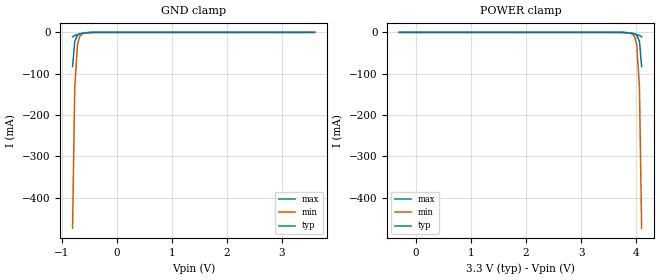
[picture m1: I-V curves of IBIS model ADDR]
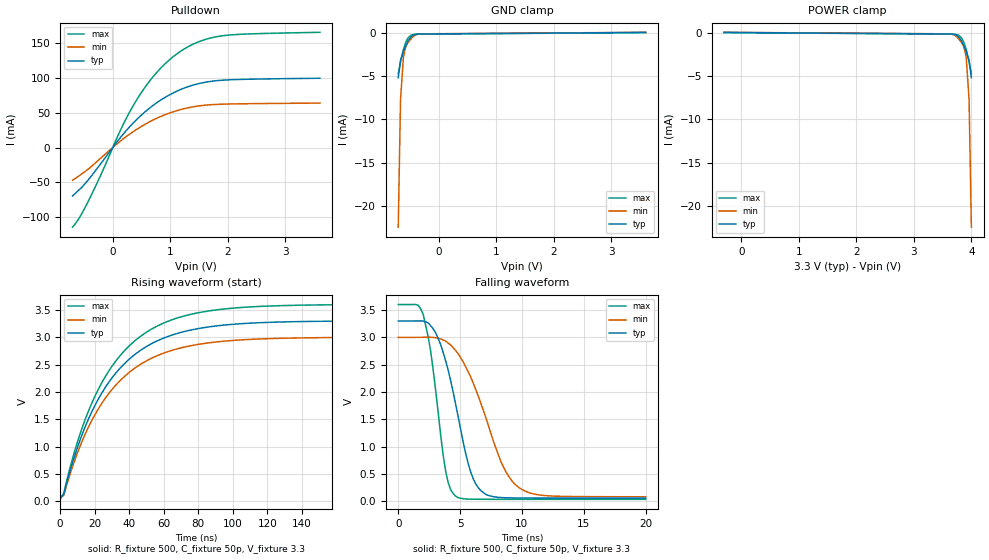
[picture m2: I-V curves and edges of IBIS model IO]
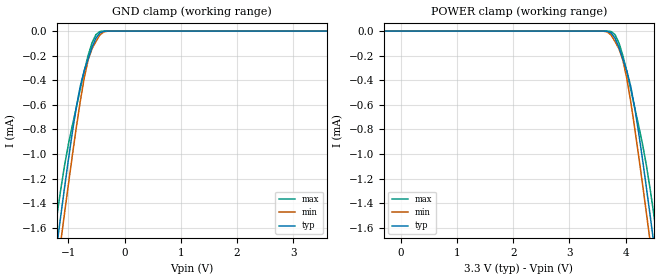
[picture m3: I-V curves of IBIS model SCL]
[IBIS Ver]   3.2
[Comment Char]   |_char
| Vnom = 3.3v, Vmin = 3v, Vmax = 3.6v
[File name]   pca8575_3_3v.ibs
[File Rev]   1
[Date]   Aug 6, 2008 4:45:34 PM
[Source]
Generated by Seshadri Venkataramanan using IBIS Toolkit at NXP Tempe
[Notes]
[Disclaimer]
(C) Copyright 2007 NXP Semiconductors
All rights reserved
NXP Semiconductors (NXP) does not warrant that this model and any other
accompanying information (Model) accurately or fully represents the
operating characteristics and specifications of the semiconductor
products to which the Model relates.  Moreover, the Model is furnished
on an "as is" and with "all faults" basis, and without support or
warranty of any kind.  NXP disclaims all warranties, whether expressed
or implied or statutory, including without limitation all implied
warranties of non-infringement, merchantability and fitness for any
purpose, and those arising from a course of dealing or usage of trade.
NXP does not convey any license under its or any third party's patents,
copyrights or other intellectual property or proprietary rights.
You and your company assume any and all risks and liability arising out
of the application or use of the Model.
In no event shall NXP be liable for any direct, indirect, special,
consequential or incidental damages, however caused, whether in
warranty, contract or tort (including negligence), strict liability or
other legal theory, including, without limitation, for lost profits,
business interruption, or corruption or loss of data or information,
arising out of or in connection with the use of or the inability to use
the Model, even if NXP has been advised of the possibility of such
damages.
NXP provides the Model as a courtesy to our customers. You and your
company shall not distribute, convey, sell, or give the Model to anyone
else without receiving prior written permission from NXP.
NXP reserves the right to make changes without notice to the Model to
improve reliability, function, or design.
Please be aware that your receipt and subsequent use of the Model shall
serve as acceptance of these terms and conditions.  If you do not
accept these terms, return or destroy the Model immediately.
[Copyright]
2008
| SO24 package
[Component]   PCA8575D
Si_location Pin
Timing_location Pin
[Manufacturer]   NXP Semiconductors
[Package]
R_pkg   0.14   0.12   0.18
L_pkg   5.71n   3.95n   7.95n
C_pkg   1.01p   0.72p   1.49p
[Pin] signal_name   model_name   R_pin   L_pin   C_pin
1   INTb   INT_OUT   0.18   6.01n   0.97p
2   AD1   ADDR   0.14   7.94n   1.21p
3   AD2   ADDR   0.16   7.06n   1.32p
4   P00   IO   0.18   6.01n   1.07p
5   P01   IO   0.14   4.98n   0.88p
6   P02   IO   0.13   4.30n   0.80p
7   P03   IO   0.12   3.95n   0.74p
8   P04   IO   0.12   3.95n   0.72p
9   P05   IO   0.13   4.30n   0.76p
10   P06   IO   0.14   4.98n   0.85p
11   P07   IO   0.18   6.01n   0.97p
12   VSS   GND   0.16   7.06n   1.20p
13   P10   IO   0.14   7.95n   1.45p
14   P11   IO   0.14   7.95n   1.49p
15   P12   IO   0.16   7.06n   1.32p
16   P13   IO   0.18   6.01n   1.07p
17   P14   IO   0.14   4.98n   0.88p
18   P15   IO   0.13   4.30n   0.80p
19   P16   IO   0.12   3.95n   0.74p
20   P17   IO   0.12   3.95n   0.72p
21   AD0   ADDR   0.13   4.30n   0.76p
22   SCL   SCL   0.14   4.98n   0.85p
23   SDA   SDAIO   0.18   6.01n   0.97p
24   VDD   POWER   0.16   7.06n   1.20p
| TSSOP24 package
[Component]   PCA8575PW
Si_location Pin
Timing_location Pin
[Manufacturer]   NXP Semiconductors
[Package]
R_pkg   52.70m   31.50m   67.00m
L_pkg   2.19n   1.32n   3.39n
C_pkg   0.48p   0.35p   0.93p
[Pin] signal_name   model_name   R_pin   L_pin   C_pin
1   INTb   INT_OUT   66.40m   2.36n   0.47p
2   AD1   ADDR   66.10m   3.39n   0.57p
3   AD2   ADDR   67.00m   2.94n   0.59p
4   P00   IO   66.40m   2.36n   0.47p
5   P01   IO   47.10m   1.67n   0.40p
6   P02   IO   38.00m   1.44n   0.37p
7   P03   IO   31.50m   1.32n   0.35p
8   P04   IO   31.50m   1.32n   0.35p
9   P05   IO   38.00m   1.44n   0.37p
10   P06   IO   47.10m   1.67n   0.40p
11   P07   IO   66.40m   2.36n   0.47p
12   VSS   GND   67.00m   2.94n   0.59p
13   P10   IO   66.10m   3.39n   0.61p
14   P11   IO   66.20m   3.39n   0.61p
15   P12   IO   67.00m   2.94n   0.59p
16   P13   IO   66.50m   2.36n   0.47p
17   P14   IO   47.10m   1.67n   0.40p
18   P15   IO   38.00m   1.45n   0.37p
19   P16   IO   31.50m   1.32n   0.35p
20   P17   IO   31.50m   1.32n   0.35p
21   AD0   ADDR   38.00m   1.45n   0.37p
22   SCL   SCL   47.10m   1.67n   0.40p
23   SDA   SDAIO   66.50m   2.36n   0.47p
24   VDD   POWER   67.00m   2.94n   0.59p
| SSOP24
[Component]   PCA8575DB
Si_location Pin
Timing_location Pin
[Manufacturer]   NXP Semiconductors
[Package]
R_pkg   54.20m   39.70m   64.80m
L_pkg   2.55n   1.89n   3.58n
C_pkg   0.636p   0.52p   1.05p
[Pin] signal_name   model_name   R_pin   L_pin   C_pin
1   INTb   INT_OUT   63.00m   2.53n   0.58p
2   AD1   ADDR   61.20m   3.56n   0.70p
3   AD2   ADDR   64.80m   3.10n   0.76p
4   P00   IO   63.00m   2.53n   0.60p
5   P01   IO   52.60m   2.17n   0.57p
6   P02   IO   43.90m   2.03n   0.56p
7   P03   IO   39.70m   1.89n   0.54p
8   P04   IO   39.70m   1.89n   0.52p
9   P05   IO   43.90m   2.03n   0.55p
10   P06   IO   52.60m   2.17n   0.56p
11   P07   IO   63.00m   2.53n   0.58p
12   VSS   GND   64.80m   3.10n   0.71p
13   P10   IO   61.20m   3.56n   1.01p
14   P11   IO   61.20m   3.56n   1.05p
15   P12   IO   64.80m   3.10n   0.80p
16   P13   IO   63.00m   2.53n   0.65p
17   P14   IO   52.60m   2.17n   0.59p
18   P15   IO   43.90m   2.03n   0.56p
19   P16   IO   39.70m   1.89n   0.54p
20   P17   IO   39.70m   1.89n   0.53p
21   AD0   ADDR   43.90m   2.03n   0.56p
22   SCL   SCL   52.60m   2.17n   0.57p
23   SDA   SDAIO   63.00m   2.53n   0.60p
24   VDD   POWER   64.80m   3.10n   0.76p
[Define Package Model]  HVQFN24
[Manufacturer]  ST-NXP Wireless
|[Simulated] Chris Hunat
|[Approved] Wayne Nunn, Roger Real
[OEM]  Unknown
[Description]  Full package model
[Number Of Pins]  23
[Pin Numbers]
pin1   | pin1 = lead1
pin2   | pin2 = lead2
pin3   | pin3 = lead3
pin4   | pin4 = lead4
pin5   | pin5 = lead5
pin6   | pin6 = lead6
pin7   | pin7 = lead7
pin8   | pin8 = lead8
pin9   | pin9 = lead9
pin10   | pin10 = lead10
pin11   | pin11 = lead11
pin12   | pin12 = lead12
pin13   | pin13 = lead13
pin14   | pin14 = lead14
pin15   | pin15 = lead15
pin17   | pin17 = lead17
pin18   | pin18 = lead18
pin19   | pin19 = lead19
pin20   | pin20 = lead20
pin21   | pin21 = lead21
pin22   | pin22 = lead22
pin23   | pin23 = lead23
pin24   | pin24 = lead24
[Model Data]
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[End Model Data]
[End Package Model]
[Define Package Model]  DHVQFN24
[Manufacturer]  ST-NXP Wireless
|[Simulated] Chris Hunat
|[Approved] Wayne Nunn, Roger Real
[OEM]  Unknown
[Description]  Full package model
[Number Of Pins]  24
[Pin Numbers]
|Pin Num   Terminal Name
1   | lead1:pin1
2   | lead2:pin2
3   | lead3:pin3
4   | lead4:pin4
5   | lead5:pin5
6   | lead6:pin6
7   | lead7:pin7
8   | lead8:pin8
9   | lead9:pin9
10   | lead10:pin10
11   | lead11:pin11
12   | lead12:pin12
13   | lead13:pin13
14   | lead14:pin14
15   | lead15:pin15
16   | lead16:pin16
17   | lead17:pin17
18   | lead18:pin18
19   | lead19:pin19
20   | lead20:pin20
21   | lead21:pin21
22   | lead22:pin22
23   | lead23:pin23
24   | lead24:pin24
[Model Data]
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[End Model Data]
[End Package Model]
| Models and submodels in the file (5): ADDR (Input), IO (I/O_open_drain), SCL (Input), SDAIO (I/O_open_drain), INT_OUT (Open_drain)
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[Model]   ADDR
Model_type Input
Vinh=2.31
Vinl=0.99
C_comp   0.73p   0.7p   0.76p
[Temperature Range] 27   85   -40
[Voltage Range]   3.3   3   3.6
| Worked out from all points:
|   GND clamp passes 1 mA (typ) near -0.54 V on its own axis
[GND Clamp]
-800mV    -82.74mA   -473.3mA   -10.75mA
-760mV    -21.49mA   -132.6mA   -7.457mA
-710mV    -6.279mA   -28.8mA    -5.482mA
-670mV    -3.609mA   -9.611mA   -3.955mA
-620mV    -2.373mA   -3.263mA   -2.228mA
-360mV    -13.44uA   -47.6uA    -1.436uA
3.6V      65.11pA    250.9pA    47.06pA
[POWER Clamp]
-300mV    65.11pA    250.9pA    47.06pA
3.66V     -13.44uA   -47.6uA    -1.436uA
3.92V     -2.373mA   -3.263mA   -2.228mA
3.97V     -3.609mA   -9.611mA   -3.955mA
4.01V     -6.279mA   -28.8mA    -5.482mA
4.06V     -21.49mA   -132.6mA   -7.457mA
4.1V      -82.74mA   -473.3mA   -10.75mA
[Model]   IO
Model_type I/O_open_drain
Vinh=2.31
Vinl=0.99
Vref=3.3
Vmeas=1.65
Rref=500
Cref=50p
C_comp   6.3p   6.1p   6.5p
[Temperature Range] 27   85   -40
[Voltage Range]   3.3   3   3.6
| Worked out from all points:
|   slope of the pulldown table from 0 to 0.495 V, typ, clamps not added: 10.7 ohm
|   GND clamp passes 1 mA (typ) near -0.53 V on its own axis
|   falling waveform, R_fixture 500, C_fixture 50p, V_fixture 3.3: 20-80 % time 1.91ns typ, 2.87ns min, 1.18ns max; typ from 3.3 V to 0.059 V
|   rising waveform, R_fixture 500, C_fixture 50p, V_fixture 3.3: 20-80 % time 34.7ns typ, 34.9ns min, 34.6ns max; typ from 0.059 V to 3.3 V
[Pulldown]
-700mV    -69.7mA    -47.05mA   -114.6mA
-570mV    -59.72mA   -39.74mA   -99.52mA
-440mV    -47.94mA   -31.96mA   -79.59mA
-220mV    -24.4mA    -16mA      -41.54mA
130mV     14.17mA    9.129mA    24.49mA
390mV     38.29mA    24.83mA    65.26mA
690mV     60.06mA    39.22mA    101mA
1.04V     78.26mA    51.25mA    130.2mA
1.43V     90.71mA    59.12mA    150.2mA
1.82V     96.42mA    62.18mA    159.9mA
2.3V      98.29mA    63.09mA    163.4mA
3.6V      99.8mA     64.04mA    165.9mA
[GND Clamp]
-700mV    -5.214mA   -22.45mA   -4.761mA
-660mV    -3.193mA   -7.746mA   -3.384mA
-610mV    -2.184mA   -2.823mA   -1.938mA
-570mV    -1.557mA   -1.664mA   -1.134mA
-530mV    -970.2uA   -1.155mA   -623.8uA
-480mV    -502.1uA   -745.6uA   -309.2uA
-440mV    -304.5uA   -449.9uA   -220.2uA
-350mV    -174.4uA   -181uA     -184.3uA
-270mV    -162.3uA   -146.3uA   -179.8uA
3.6V      13.62uA    27.33uA    109.1pA
[POWER Clamp]
-300mV    13.62uA    27.33uA    109.1pA
3.57V     -162.3uA   -146.3uA   -179.8uA
3.65V     -174.4uA   -181uA     -184.3uA
3.74V     -304.5uA   -449.9uA   -220.2uA
3.78V     -502.1uA   -745.6uA   -309.2uA
3.83V     -970.2uA   -1.155mA   -623.8uA
3.87V     -1.557mA   -1.664mA   -1.134mA
3.91V     -2.184mA   -2.823mA   -1.938mA
3.96V     -3.193mA   -7.746mA   -3.384mA
4V        -5.214mA   -22.45mA   -4.761mA
[Falling Waveform]
R_fixture=500
C_fixture=50p
V_fixture=3.3
V_fixture_min=3
V_fixture_max=3.6
0s        3.3V       3V         3.6V
2.02ns    3.299V     3.001V     3.418V
2.626ns   3.212V     3.001V     2.736V
3.838ns   2.566V     2.93V      546.6mV
4.646ns   1.77V      2.757V     94.01mV
5.657ns   689.7mV    2.37V      40.11mV
6.263ns   319.8mV    2.046V     38.13mV
8.283ns   69.49mV    735.7mV    36.84mV
9.697ns   61.34mV    261.2mV    36.7mV
20ns      58.61mV    83.49mV    36.65mV
[Rising Waveform]
R_fixture=500
C_fixture=50p
V_fixture=3.3
V_fixture_min=3
V_fixture_max=3.6
0s        58.6mV     83.02mV    36.65mV
2.02ns    121.8mV    105mV      141.7mV
8.081ns   801.2mV    718.2mV    884.1mV
14.14ns   1.337V     1.205V     1.468V
24.24ns   1.987V     1.798V     2.176V
36.36ns   2.49V      2.258V     2.724V
52.53ns   2.876V     2.61V      3.142V
70.71ns   3.095V     2.811V     3.379V
96.97ns   3.228V     2.934V     3.523V
200ns     3.299V     2.999V     3.599V
[Ramp]
R_load=500
dV/dt_r   4.390E-2/1.249E-9   3.873E-2/1.453E-9   4.900E-2/1.041E-9
dV/dt_f   1.945E+0/5.219E-10   1.750E+0/9.146E-10   2.138E+0/2.739E-10
|[End   IO
[Model]   SCL
Model_type Input
Vinh=2.31
Vinl=0.99
C_comp   2.1p   1.9p   2.3p
[Temperature Range] 27   85   -40
[Voltage Range]   3.3   3   3.6
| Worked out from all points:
|   GND clamp passes 1 mA (typ) near -0.99 V on its own axis
[GND Clamp]
-3.3V     -9.437mA   -9.646mA   -9.167mA
-1.28V    -2.005mA   -2.221mA   -1.754mA
-1.21V    -1.759mA   -1.973mA   -1.521mA
-1.14V    -1.515mA   -1.727mA   -1.299mA
-1.07V    -1.277mA   -1.484mA   -1.096mA
-930mV    -823.1uA   -1.011mA   -767.3uA
-790mV    -449.8uA   -573.6uA   -472.3uA
-650mV    -228.6uA   -236.2uA   -199.5uA
-510mV    -56.75uA   -84.45uA   -28.37uA
-440mV    -14.75uA   -31.48uA   -3.492uA
-230mV    -8.293nA   -57.44nA   -265.7pA
3.6V      8.544pA    24.57pA    7.213pA
[POWER Clamp]
-300mV    8.544pA    24.57pA    7.213pA
3.53V     -8.293nA   -57.44nA   -265.7pA
3.74V     -14.75uA   -31.48uA   -3.492uA
3.81V     -56.75uA   -84.45uA   -28.37uA
3.95V     -228.6uA   -236.2uA   -199.5uA
4.09V     -449.8uA   -573.6uA   -472.3uA
4.23V     -823.1uA   -1.011mA   -767.3uA
4.37V     -1.277mA   -1.484mA   -1.096mA
4.44V     -1.515mA   -1.727mA   -1.299mA
4.51V     -1.759mA   -1.973mA   -1.521mA
4.58V     -2.005mA   -2.221mA   -1.754mA
6.6V      -9.437mA   -9.646mA   -9.167mA
